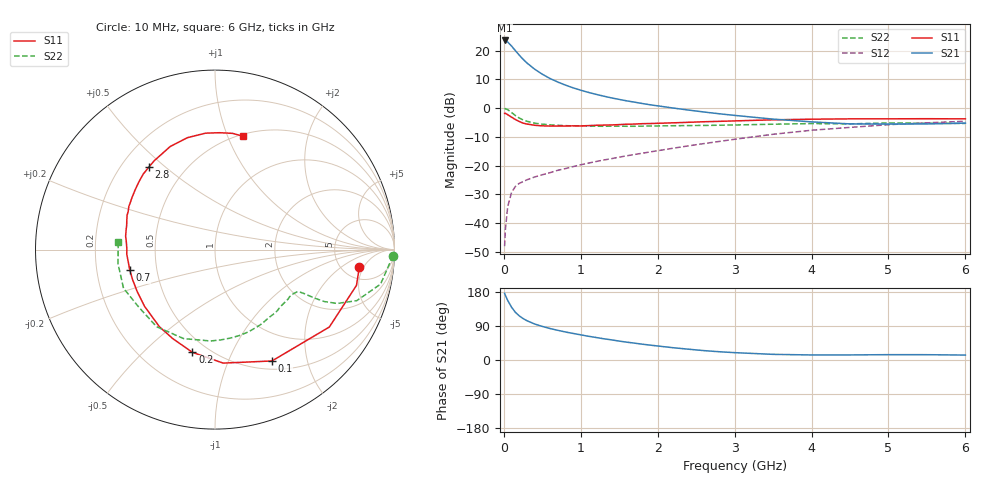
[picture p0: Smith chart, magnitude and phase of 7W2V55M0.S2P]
! Infineon Technologies  Discrete & RF Semiconductors
! BFS17W
! Si NPN RF Bipolar Junction Transistor in SOT323
! VCE = 2.5 V  IC = 5 mA
! Common Emitter S-Parameters:  August  1999
# GHz  S  MA  R  50
!  f  S11  S21  S12  S22
! GHz  MAG  ANG  MAG  ANG  MAG  ANG  MAG  ANG
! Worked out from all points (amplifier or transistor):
!   36 points, 10 MHz to 6 GHz, reference 50 ohm
!   highest |S21| = 23.5 dB at 10 MHz (marker M1)
!   |S21| within 3 dB of that: start of sweep to 133.3 MHz
!   unconditionally stable (mu >= 1): 540.8 MHz to 3.099 GHz; 4.074 GHz to end of sweep
!   at 250 MHz: K = 0.60, MSG = 21.2 dB, |S12| = -25.5 dB
!   at 1.4 GHz: K = 1.27, MAG = 7.4 dB, |S12| = -17.6 dB
!   at 6 GHz: K = 1.09, MAG = -2.2 dB, |S12| = -4.6 dB
!   S11 on the Smith chart (normalised r, x): 10 MHz: 7.19, -4.07; 100 MHz: 0.60, -1.46; 200 MHz: 0.41, -0.72; 700 MHz: 0.35, -0.10; 2.8 GHz: 0.31, +0.44; 6 GHz: 0.52, +1.13
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0.01  0.8101 -6.9  14.98 175.9  0.004 85.2  0.9931 -2.0
0.02  0.8131 -14.2  14.97 170.6  0.0077 84.9  0.9739 -4.9
0.05  0.7693 -34.1  14.07 157.3  0.0194 74.6  0.9421 -11.8
0.1  0.697 -62.9  11.99 139.4  0.0342 61.0  0.8396 -19.8
0.15  0.634 -85.9  9.969 125.9  0.0436 53.3  0.7439 -23.8
0.2  0.586 -102.4  8.339 116.5  0.0493 49.9  0.6747 -25.4
0.25  0.5491 -115.3  7.054 109.4  0.0529 47.1  0.6244 -25.9
0.3  0.5297 -125.8  6.09 103.7  0.0568 46.8  0.5918 -26.1
0.4  0.5038 -141.3  4.753 95.0  0.0637 47.4  0.5486 -26.3
0.5  0.4923 -151.9  3.883 88.6  0.0696 49.1  0.5274 -26.6
0.6  0.4887 -160.0  3.272 83.1  0.0756 51.2  0.5123 -27.5
0.7  0.4883 -166.5  2.845 78.4  0.0832 53.3  0.5034 -28.9
0.9  0.4923 -177.0  2.252 70.1  0.0963 55.9  0.4912 -32.4
1.1  0.4967 174.5  1.876 62.6  0.1109 57.9  0.4875 -36.9
1.3  0.5073 167.4  1.612 56.0  0.1258 59.5  0.4837 -42.0
1.6  0.5257 158.7  1.335 47.0  0.1487 61.5  0.4837 -49.9
2.2  0.5552 143.4  1.004 32.4  0.2011 63.4  0.4946 -67.7
2.8  0.589 128.9  0.798 21.8  0.2639 62.4  0.5045 -86.7
3.5  0.6263 113.5  0.644 14.9  0.3513 57.8  0.5258 -109.4
4.5  0.6508 94.7  0.532 13.4  0.4625 45.8  0.5322 -143.0
5.5  0.6549 81.4  0.531 14.0  0.5552 33.5  0.5461 -171.6
6  0.6507 76.3  0.549 13.0  0.5913 27.6  0.5409 175.7
